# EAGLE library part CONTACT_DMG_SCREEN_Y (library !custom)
The vertical input for the DMG screen.
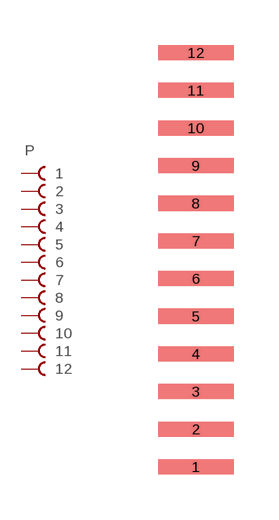
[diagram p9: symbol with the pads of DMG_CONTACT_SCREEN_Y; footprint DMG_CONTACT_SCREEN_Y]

Designator prefix P

## CONTACT_DMG_SCREEN_Y  [DMG_CONTACT_SCREEN_Y]
1  1  pas
2  2  pas
3  3  pas
4  4  pas
5  5  pas
6  6  pas
7  7  pas
8  8  pas
9  9  pas
10  10  pas
11  11  pas
12  12  pas

## Footprint DMG_CONTACT_SCREEN_Y (pad centres in mm)
smd 2.5 x 0.5: 1 0,-6.875; 2 0,-5.625; 3 0,-4.375; 4 0,-3.125; 5 0,-1.875; 6 0,-0.625; 7 0,0.625; 8 0,1.875; 9 0,3.125; 10 0,4.375; 11 0,5.625; 12 0,6.875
